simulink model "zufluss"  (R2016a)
settings: Solver=ode45  StartTime=0.0  StopTime=10.0  MaxStep=1  RelTol=1e-3
undefined symbols (not defined in the file or in its folder): k, m0

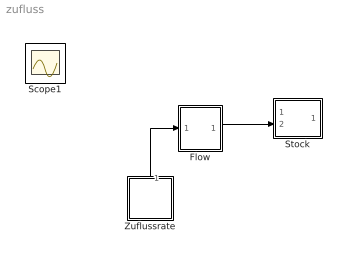
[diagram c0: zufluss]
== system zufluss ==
  Flow : Subsystem
  Stock : Subsystem
  Zuflussrate : Subsystem
  Scope1 : Scope
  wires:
  Zuflussrate/1(Out1) -> Flow/1(In1)
  Flow/1(Out1) -> Stock/2(In2)

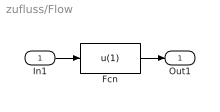
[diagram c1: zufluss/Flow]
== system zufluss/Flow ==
  In1 : Inport
  Fcn : Fcn  Expr=u(1)
  Out1 : Outport
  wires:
  In1/1 -> Fcn/1
  Fcn/1 -> Out1/1

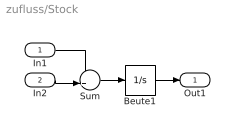
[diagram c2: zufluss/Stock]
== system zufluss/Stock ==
  In1 : Inport
  In2 : Inport  Port=2
  Beute1 : Integrator  InitialCondition=m0
  Sum : Sum  Inputs=-+|
  Out1 : Outport
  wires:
  Sum/1 -> Beute1/1
  In1/1 -> Sum/1
  Beute1/1 -> Out1/1
  In2/1 -> Sum/2

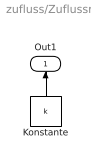
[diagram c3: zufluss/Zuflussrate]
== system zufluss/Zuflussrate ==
  Konstante : Constant  Value=k
  Out1 : Outport
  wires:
  Konstante/1 -> Out1/1
